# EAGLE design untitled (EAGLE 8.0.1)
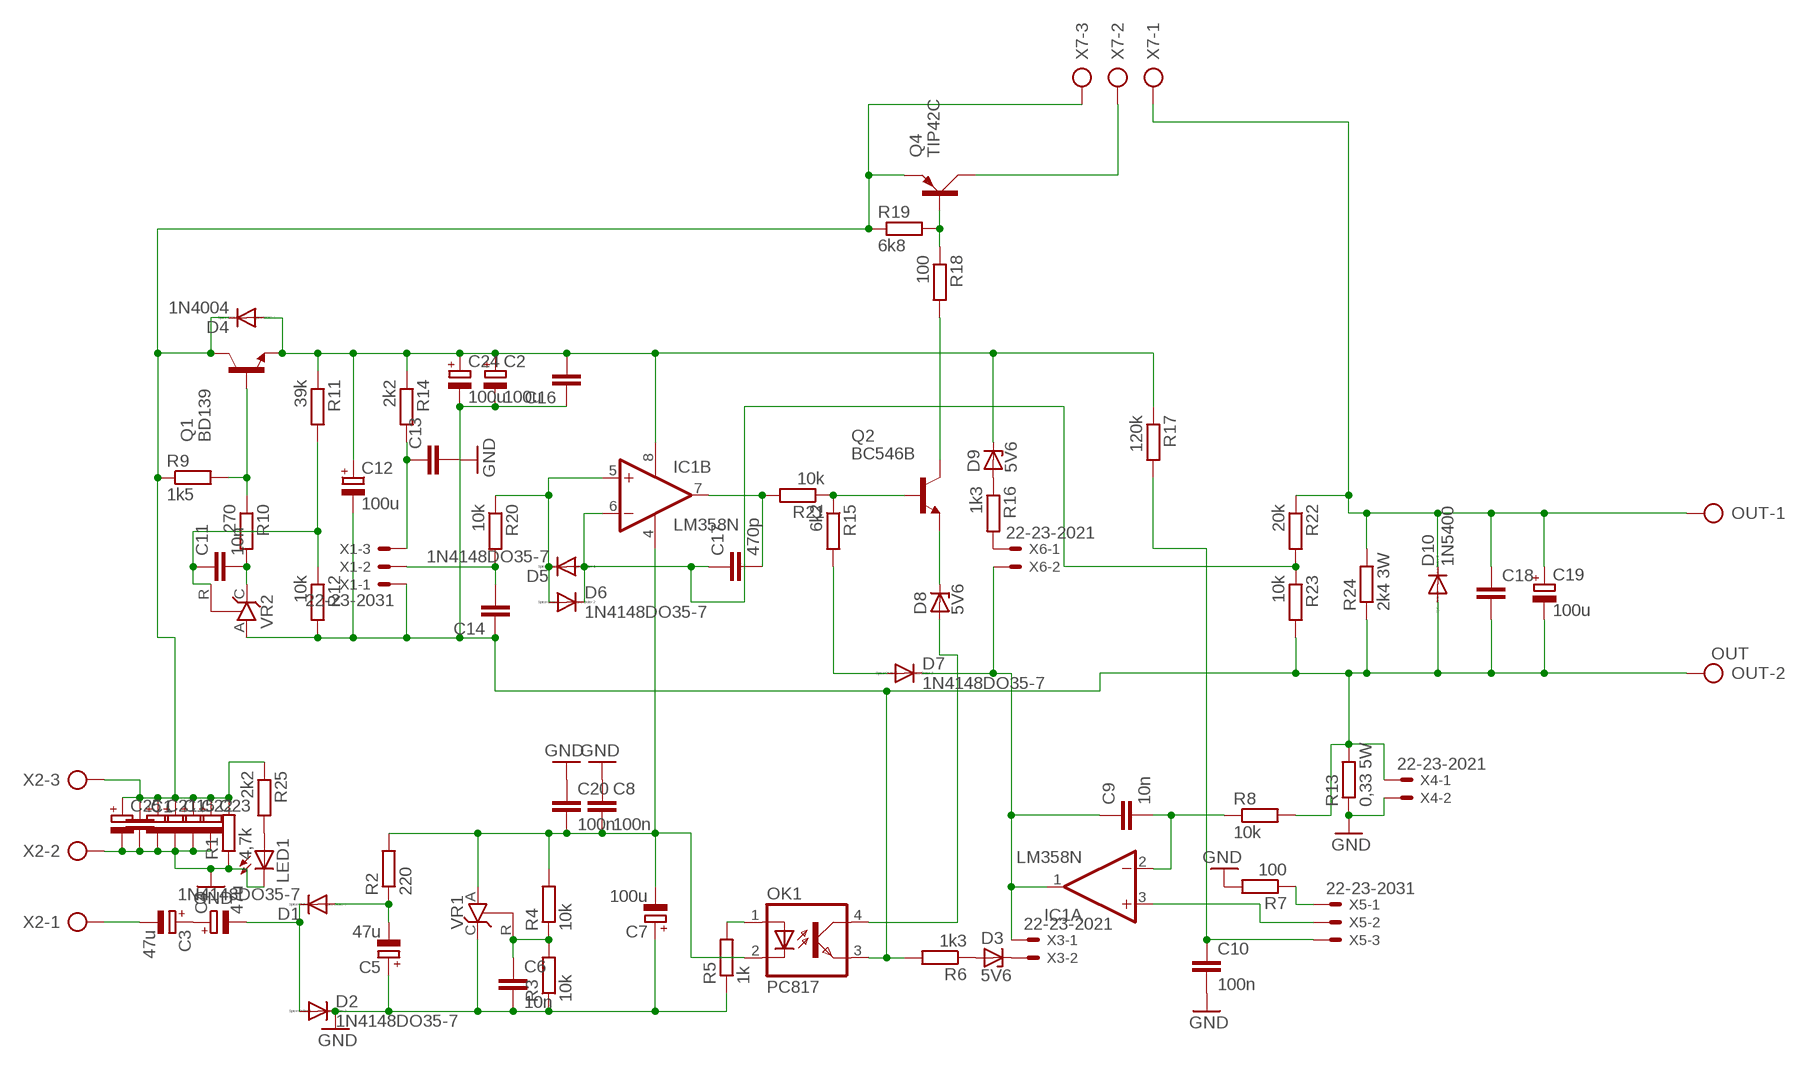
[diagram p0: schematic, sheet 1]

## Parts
C1  C-EU050-025X075  [C050-025X075]
C2  100u  CPOL-EUE2.5-7  [E2,5-7]
C3  47u  CPOL-EUE2.5-7  [E2,5-7]
C4  47u  CPOL-EUE2.5-7  [E2,5-7]
C5  47u  CPOL-EUE2.5-7  [E2,5-7]
C6  10n  C-EU050-025X075  [C050-025X075]
C7  100u  CPOL-EUE2.5-7  [E2,5-7]
C8  100n  C-EU050-025X075  [C050-025X075]
C9  10n  C-EU050-025X075  [C050-025X075]
C10  100n  C-EU050-025X075  [C050-025X075]
C11  10n  C-EU050-025X075  [C050-025X075]
C12  100u  CPOL-EUE2.5-7  [E2,5-7]
C13  C-EU050-025X075  [C050-025X075]
C14  C-EU050-025X075  [C050-025X075]
C15  CPOL-EUE5-10.5  [E5-10,5]
C16  C-EU050-025X075  [C050-025X075]
C17  470p  C-EU050-025X075  [C050-025X075]
C18  C-EU050-025X075  [C050-025X075]
C19  100u  CPOL-EUE2.5-7  [E2,5-7]
C20  100n  C-EU050-025X075  [C050-025X075]
C21  CPOL-EUE5-10.5  [E5-10,5]
C22  CPOL-EUE5-10.5  [E5-10,5]
C23  CPOL-EUE5-10.5  [E5-10,5]
C24  100u  CPOL-EUE2.5-7  [E2,5-7]
C25  CPOL-EUE5-10.5  [E5-10,5]
D1  1N4148DO35-7  [DO35-7]
D2  1N4148DO35-7  [DO35-7]
D3  5V6  BZD23  [SOD81]
D4  1N4004  [DO41-10]
D5  1N4148DO35-7  [DO35-7]
D6  1N4148DO35-7  [DO35-7]
D7  1N4148DO35-7  [DO35-7]
D8  5V6  BZD23  [SOD81]
D9  5V6  BZD23  [SOD81]
D10  1N5400  [DO201-15]
IC1  LM358N  [DIL08]
LED1  LED3MM  [LED3MM]
OK1  PC817  [DIL04]
OUT  OUT  AK300/2  [AK300/2]
Q1  BD139  [TO126]
Q2  BC546B  [TO92-EBC]
Q4  TIP42C  [TO220AV]
R1  4,7k  R-EU_0309/12  [0309/12]
R2  220  R-EU_0207/2V  [0207/2V]
R3  10k  R-EU_0207/7  [0207/7]
R4  10k  R-EU_0207/2V  [0207/2V]
R5  1k  R-EU_0207/7  [0207/7]
R6  1k3  R-EU_0207/7  [0207/7]
R7  100  R-EU_0207/7  [0207/7]
R8  10k  R-EU_0207/7  [0207/7]
R9  1k5  R-EU_0207/2V  [0207/2V]
R10  270  R-EU_0207/7  [0207/7]
R11  39k  R-EU_0207/7  [0207/7]
R12  10k  R-EU_0207/2V  [0207/2V]
R13  0,33 5W  R-EU_0922/22  [0922/22]
R14  2k2  R-EU_0207/2V  [0207/2V]
R15  6k2  R-EU_0207/2V  [0207/2V]
R16  1k3  R-EU_0207/2V  [0207/2V]
R17  120k  R-EU_0204/5  [0204/5]
R18  100  R-EU_0207/10  [0207/10]
R19  6k8  R-EU_0207/7  [0207/7]
R20  10k  R-EU_0207/2V  [0207/2V]
R21  10k  R-EU_0207/7  [0207/7]
R22  20k  R-EU_0207/10  [0207/10]
R23  10k  R-EU_0207/7  [0207/7]
R24  2k4 3W  R-EU_0309/12  [0309/12]
R25  2k2  R-EU_0207/2V  [0207/2V]
VR1  TL431CLP  [TO92-CLP]
VR2  TL431CLP  [TO92-CLP]
X1  22-23-2031  [22-23-2031]
X2  AK300/3  [AK300/3]
X3  22-23-2021  [22-23-2021]
X4  22-23-2021  [22-23-2021]
X5  22-23-2031  [22-23-2031]
X6  22-23-2021  [22-23-2021]
X7  AK300/3  [AK300/3]

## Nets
GND: C1.2 C5.+ C6.2 C7.+ C8.1 C10.2 C13.2 C15.- C20.1 C21.- C22.- C23.- C25.- D2.C LED1.K(C) R1.1 R3.1 R5.1 R7.2 R13.1 VR1.C X2.2 X4.2
N$1: C1.1 C15.+ C21.+ C22.+ C23.+ C25.+ D4.C Q1.2(C) Q4.E R1.2 R9.1 R19.1 R25.1 X2.3 X7.3
N$2: C7.- C8.2 C20.2 IC1.4(P:V-) OK1.2(C) R2.2 R4.2 VR1.A
N$3: C3.+ C4.+
N$4: C3.- X2.1
N$5: C4.- D1.C D2.A
N$6: C6.1 R3.2 R4.1 VR1.R
N$7: C5.- D1.A R2.1
N$8: C2.- C12.- C14.1 C16.1 C18.2 C19.- C24.- D10.A OK1.3(EMIT) OUT.2 R6.2 R8.2 R12.2 R13.2 R23.2 R24.1 VR2.A X1.1 X4.1
N$9: D3.A R6.1
N$10: OK1.1(A) R5.2
N$11: D3.C X3.2
N$12: C9.1 D7.C IC1.1(A:OUT) X3.1 X6.2
N$13: C9.2 IC1.2(A:-IN) R8.1
N$14: C10.1 R17.2 X5.3
N$15: IC1.3(A:+IN) X5.2
N$16: R7.1 X5.1
N$18: R16.2 X6.1
N$19: C2.+ C12.+ C16.2 C24.+ D4.A D9.C IC1.8(P:V+) Q1.1(E) R11.1 R14.1 R17.1
N$20: Q1.3(B) R9.2 R10.1
N$21: C11.2 R10.2 VR2.C
N$22: C11.1 R11.2 R12.1 VR2.R
N$24: C13.1 R14.2 X1.3
N$25: C14.2 R20.2 X1.2
N$26: D9.A R16.1
N$27: D5.C D6.A IC1.5(B:+IN) R20.1
N$29: C17.2 IC1.7(B:OUT) R21.2
N$30: Q2.B R15.1 R21.1
N$31: D7.A R15.2
N$32: D8.C Q2.E
N$33: D8.A OK1.4(COL)
N$37: Q4.B R18.1 R19.2
N$38: Q2.C R18.2
N$40: Q4.C X7.2
N$41: C18.1 C19.+ D10.C OUT.1 R22.1 R24.2 X7.1
N$42: C17.1 D5.A D6.C IC1.6(B:-IN) R22.2 R23.1
N$158: LED1.A R25.2

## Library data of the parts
C1 C6 C8-C11 C13 C14 C16-C18 C20 = resistor:C-EU: CAPACITOR, European symbol
C2-C5 C7 C12 C15 C19 C21-C25 = resistor:CPOL-EU: POLARIZED CAPACITOR, European symbol
D1 D2 D5-D7 = diode:1N4148: DIODE
D3 D8 D9 = diode:BZD23: Z DIODE
D4 = diode:1N4004: DIODE
D10 = diode:1N5400: DIODE
IC1 = linear:LM358: OP AMP also LM158; LM258; LM2904 Source: http://cache.national.com/ds/LM/LM158.pdf
LED1 = led:LED: LED
OK1 = optocoupler:PC817: SHARP OPTO COUPLER; MPN: PC817X4J000F; OC_FARNELL: 9707727; OC_NEWARK: 97K7059
OUT = con-ptr500:AK300/2: CONNECTOR; OC_FARNELL: unknown; OC_NEWARK: unknown
Q1 = transistor-npn:BD139*: NPN Transistor
Q2 = transistor-npn:BC546*: NPN Transistor
Q4 = transistor-power:TIP42C: PNP TRANSISTOR
R1-R25 = resistor:R-EU_: RESISTOR, European symbol
VR1 VR2 = v-reg:TL431CLP: VOLTAGE REGULATOR
X1 X5 = con-molex:22-23-2031: .100" (2.54mm) Center Header - 3 Pin; MF: MOLEX; MPN: 22-23-2031; OC_FARNELL: 1462950; OC_NEWARK: 30C0862
X2 X7 = con-ptr500:AK300/3: CONNECTOR; OC_FARNELL: unknown; OC_NEWARK: unknown
X3 X4 X6 = con-molex:22-23-2021: .100" (2.54mm) Center Header - 2 Pin; MF: MOLEX; MPN: 22-23-2021; OC_FARNELL: 1462926; OC_NEWARK: 25C3832

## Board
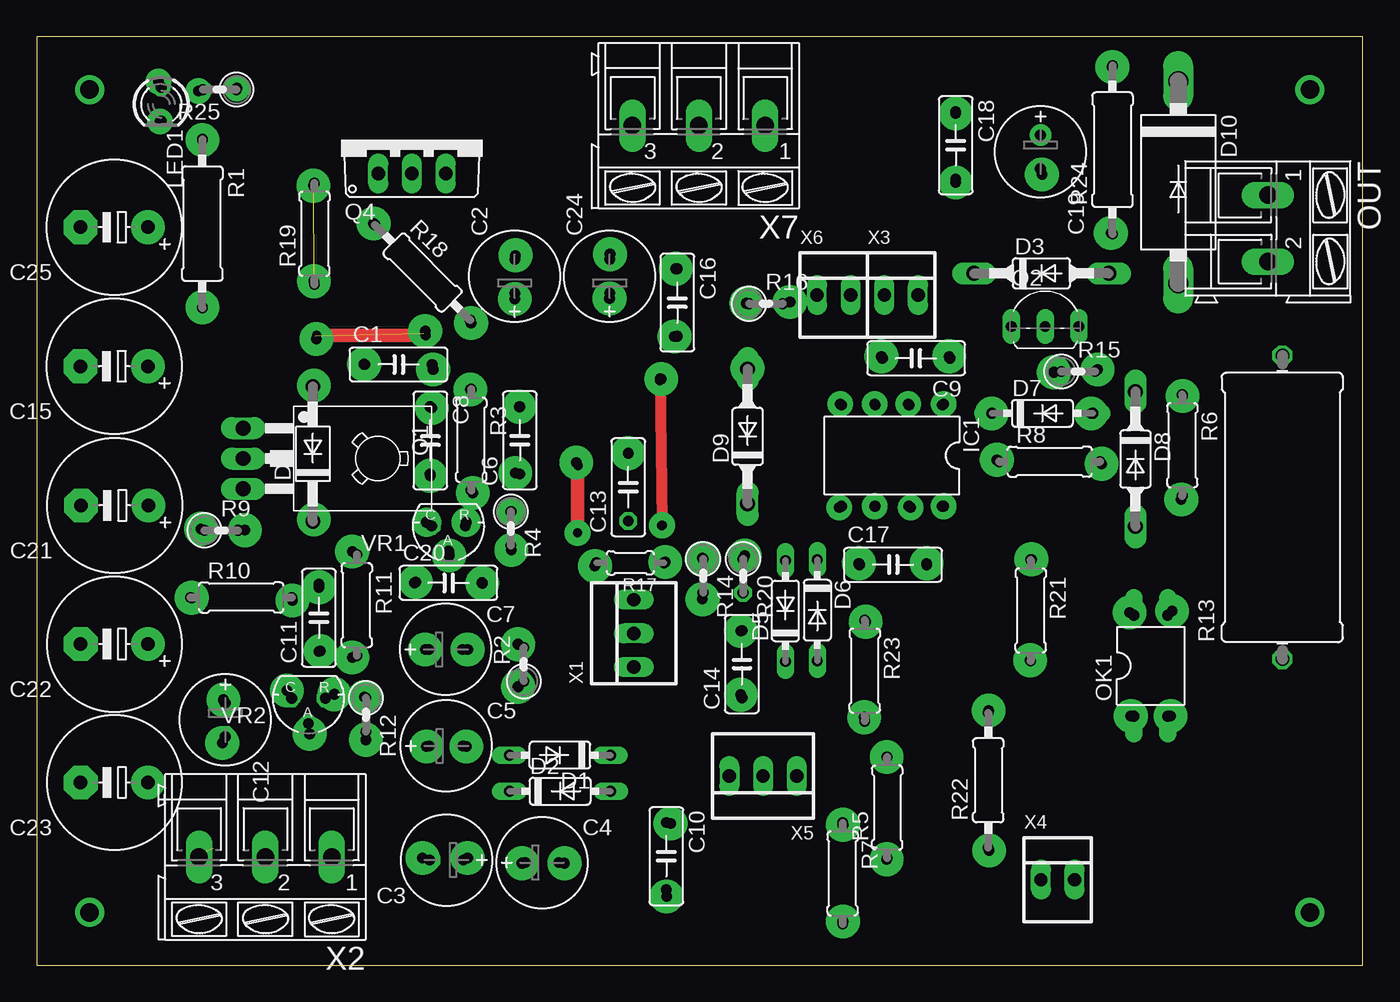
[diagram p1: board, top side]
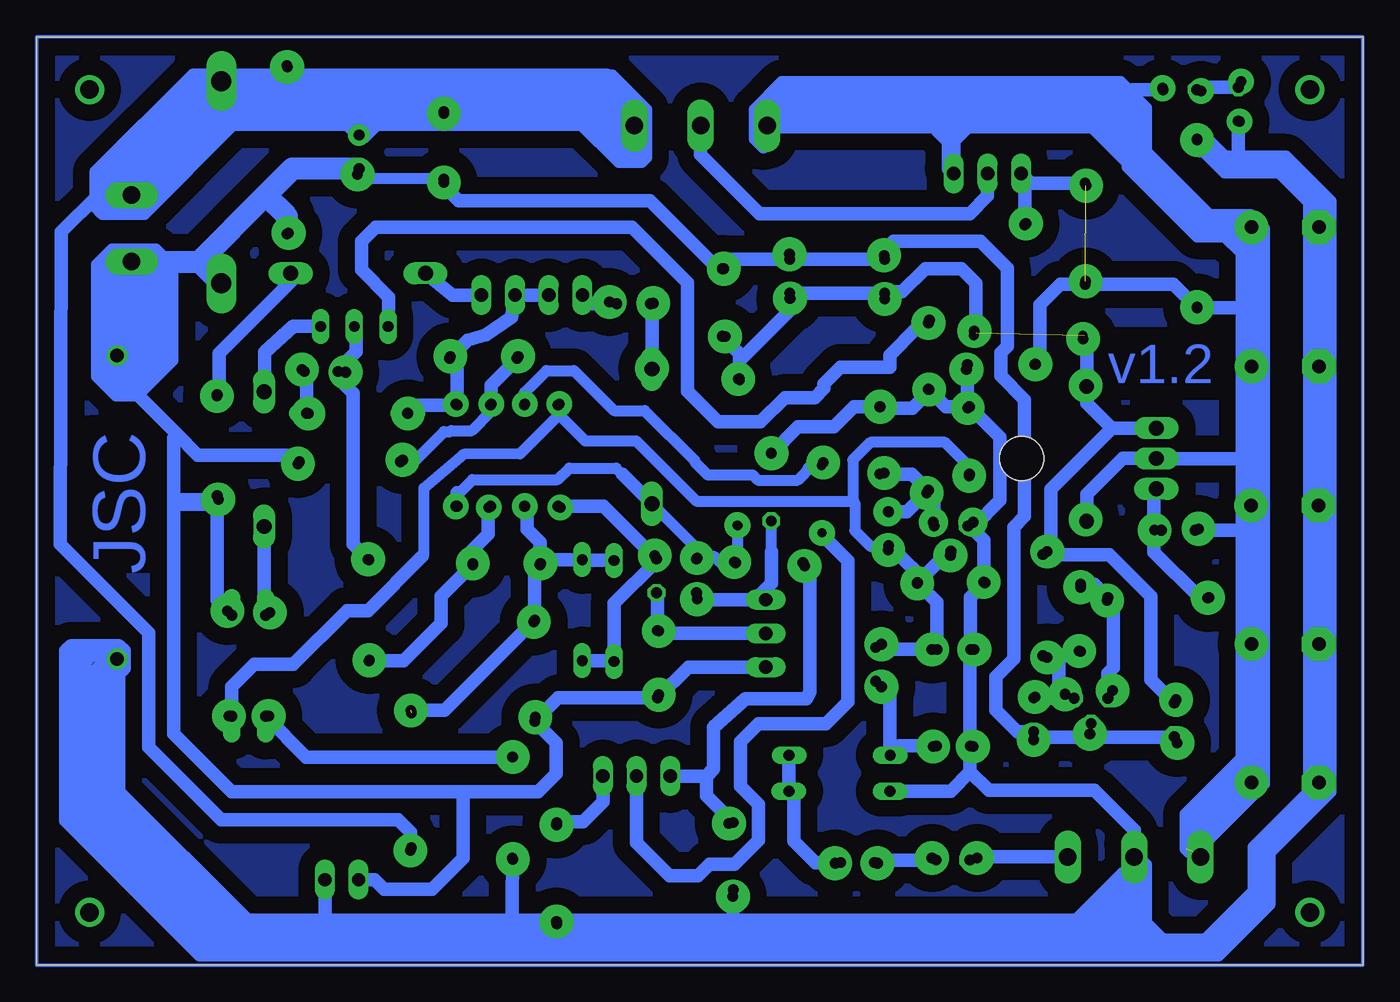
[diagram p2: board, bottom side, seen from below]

Size 100 x 70 mm. Coordinates in mm from the lower left corner, seen from the top.
Outline: 0,0 100,0 100,70 0,70 0,0
Copper layers (1*16): Top 0.035mm / dielectric 1.5mm / Bottom 0.035mm
Design rules "default": minimum track width 10mil, minimum drill 24mil, track to track 8mil, track to pad 8mil, pad to pad 8mil, via to via 8mil, smd to smd 8mil, copper to edge 40mil, drill to drill 8mil, minimum pad ring 10mil, minimum via ring 8mil, stop-mask expansion 4mil, vias tented up to drill 0mil, thermal gap 10mil

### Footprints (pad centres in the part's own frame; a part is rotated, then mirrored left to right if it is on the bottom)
C050-025X075 = drill 0.813 octagon: 1 -2.54,0; 2 2.54,0
E2,5-7 = drill 0.813 pad 1.6: + -1.27,0 | drill 0.813 pad 1.6 octagon: - 1.27,0
E5-10,5 = drill 1.016 pad 2.54: + -2.54,0 | drill 1.016 pad 2.54 octagon: - 2.54,0
DO35-7 = drill 0.813 long: A 3.81,0; C -3.81,0
SOD81 = drill 1.118 long: A 5.08,0; C -5.08,0
DO41-10 = drill 1.118: A 5.08,0; C -5.08,0
DO201-15 = drill 1.499 long: A 7.62,0; C -7.62,0
DIL08 = drill 0.813 pad 1.27: 1 -3.81,-3.81; 2 -1.27,-3.81; 3 1.27,-3.81; 4 3.81,-3.81; 5 3.81,3.81; 6 1.27,3.81; 7 -1.27,3.81; 8 -3.81,3.81
LED3MM = drill 0.813 octagon: A -1.27,0; K 1.27,0
DIL04 = drill 0.813 offset: 1 -1.27,-3.81; 2 1.27,-3.81; 3 1.27,3.81; 4 -1.27,3.81
AK300/2 = drill 1.321 long: 1 -2.515,0; 2 2.489,0
TO126 = drill 1.118 long: 1 -2.286,-5.08; 2 0,-5.08; 3 2.286,-5.08 | hole 3.302: 0,5.08
TO92-EBC = drill 0.813 long: B 0,-1.27; C -2.54,-1.27; E 2.54,-1.27
TO220AV = drill 1.016 long: B -2.54,-2.54; C 0,-2.54; E 2.54,-2.54
0309/12 = drill 0.813 octagon: 1 -6.35,0; 2 6.35,0
0207/2V = drill 0.813 octagon: 1 -1.27,0; 2 1.27,0
0207/7 = drill 0.813 octagon: 1 -3.81,0; 2 3.81,0
0922/22 = drill 1.016 octagon: 1 -11.43,0; 2 11.43,0
0204/5 = drill 0.813 octagon: 1 -2.54,0; 2 2.54,0
0207/10 = drill 0.813 octagon: 1 -5.08,0; 2 5.08,0
TO92-CLP = drill 0.813 octagon: A 0,1.905; C 1.27,0; R -1.27,0
22-23-2031 = drill 1 long: 1 -2.54,0; 2 0,0; 3 2.54,0
AK300/3 = drill 1.321 long: 1 -5.004,0; 2 0,0; 3 5.004,0
22-23-2021 = drill 1 long: 1 -1.27,0; 2 1.27,0

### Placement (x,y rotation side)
C1  27.29,45.29 0 top
C2  36.05,51.93 90 top
C3  30.9,7.94 180 top
C4  38.11,7.75 0 top
C5  30.89,16.54 0 top
C6  36.44,39.57 90 top
C7  30.85,23.81 0 top
C8  29.68,39.56 270 top
C9  66.31,45.75 180 top
C10  47.48,8.23 270 top
C11  21.29,26.19 90 top
C12  14.23,18.5 270 top
C13  44.61,36.03 90 top
C14  53.18,22.7 90 top
C15  5.85,45.15 180 top
C16  48.31,49.95 270 top
C17  64.57,30.2 0 top
C18  69.3,61.81 270 top
C19  75.69,61.31 270 top
C20  31.05,28.83 0 top
C21  5.9,34.66 180 top
C22  5.87,24.21 180 top
C23  5.87,13.78 180 top
C24  43.21,51.94 90 top
C25  5.86,55.63 180 top
D1  39.46,15.84 180 top
D2  39.47,13.13 0 top
D3  75.76,52.16 0 top
D4  20.83,38.55 90 top
D5  56.46,26.71 90 top
D6  58.86,26.77 270 top
D7  75.83,41.61 0 top
D8  82.84,38.16 270 top
D9  53.61,39.87 90 top
D10  86.07,59.02 270 top
IC1  64.49,38.42 180 top
LED1  9.4,64.9 270 top
OK1  84,22.58 0 top
OUT  92.83,55.53 270 top
Q1  20.65,38.2 270 top
Q2  76.04,49.42 0 top
Q4  28.3,62.22 0 top
R1  12.5,55.9 270 top
R2  36.73,22.69 90 top
R3  32.77,39.61 270 top
R4  35.75,32.92 270 top
R5  64.13,11.89 90 top
R6  86.38,39.2 270 top
R7  60.77,6.93 270 top
R8  76.38,37.96 0 top
R9  13.93,32.79 0 top
R10  15.43,27.73 0 top
R11  24.14,27.15 270 top
R12  24.83,18.88 270 top
R13  93.92,34.52 90 top
R14  50.25,29.36 270 top
R15  78.53,44.76 0 top
R16  54.99,49.87 0 top
R17  44.76,30.34 180 top
R18  29.1,52.22 315 top
R19  20.95,55.14 90 top
R20  53.26,29.35 270 top
R21  74.95,26.75 270 top
R22  71.75,13.95 90 top
R23  62.44,22.21 270 top
R24  81.12,61.47 90 top
R25  13.8,66 180 top
VR1  31.06,33.11 180 top
VR2  20.5,20.13 180 top
X1  45.03,25.02 90 top
X2  17.25,8.17 180 top
X3  65.19,50.52 0 top
X4  76.99,6.46 0 top
X5  54.77,14.27 180 top
X6  60.11,50.52 0 top
X7  49.93,63.28 180 top

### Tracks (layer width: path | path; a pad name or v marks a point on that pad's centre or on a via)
GND
  Bottom 1.016: 29.62,14.59 28.22,13.19 20.26,13.19 17.25,10.18 X2.2 17.25,7.47 | C8.1 27.37,39.79 27.37,35.04 29.3,33.11 VR1.C 29.63,33.11 28.57,32.05 28.57,28.89 C20.1 29.58,27.76 C7.+ 29.62,23.77 C5.+ 29.62,14.59 | C8.1 31.45,42.1 R3.1 32.77,43.2 33.97,42 36.33,42 C6.2 | C6.2 36.44,42.09 | 17.25,7.47 17.25,5.27 21.23,1.29 47.42,1.29 | 61.02,1.29 47.42,1.29 | 64.49,1.29 61.02,1.29 | 78.49,1.29 64.49,1.29 | 78.49,1.29 84.59,1.29 95.11,12 95.17,21.84 R13.1 | C10.2 47.48,1.35 47.42,1.29 | R7.2 60.77,1.54 61.02,1.29 | R5.1 64.18,1.6 64.49,1.29 | 17.25,7.47 17.29,7.43 17.29,2.92 15.55,1.18 11.74,1.18 8.1,4.82 8.1,8.84 3.32,13.62 C23.- 3.32,27.29 C22.- 3.22,37.87 C21.- 3.17,47.99 | C1.2 29.83,42.25 C8.1 | D2.C 31.08,13.13 29.62,14.59 | C13.2 42.58,40.6 39.89,40.6 38.38,42.11 C6.2 | 3.17,47.99 3.17,48.58 C15.- | 3.17,47.99 3.06,48.1 C25.- 3.32,57.69 5.84,60.21 8.9,60.21 | 8.9,60.21 10.46,60.21 R1.1 | LED1.K 9.4,60.71 8.9,60.21 | X4.2 78.26,1.52 78.49,1.29
N$1
  Bottom 1.016: D4.C 20.83,35.49 18.09,38.23 15.6,38.23 Q1.2 8.49,38.2 8.25,38.44 | X2.3 11.98,8.44 11.98,10.25 8.4,13.83 C23.+ 8.4,27.29 C22.+ 8.3,32.62 | 18.79,64.58 24.62,64.58 | 24.79,64.41 24.62,64.58 | X7.3 43.63,64.58 31.01,64.58 | 31.01,64.58 24.62,64.58 | 8.25,38.44 C21.+ 8.3,37.87 8.3,32.62 | 8.25,38.44 8.25,48.58 C15.+ 8.26,49.6 | 8.26,49.6 8.21,51.15 8.21,55.44 C25.+ 8.55,55.48 12.21,55.48 16.84,60.11 16.84,61.32 18.79,63.27 18.79,64.58 | R9.1 8.47,32.79 8.3,32.62 | 8.26,49.6 8.31,49.55 R1.2 14.28,51.33 R19.1 22.82,51.33 24.35,49.8 24.35,45.69 C1.1 | R25.1 17.37,66 18.79,64.58 | 31.01,64.58 31.01,59.85 Q4.E 30.84,62.14 29.91,63.07 29.91,63.48 31.01,64.58
N$2
  Bottom 0.813: 70.94,30.82 70.81,30.95 70.81,35.96 67.82,38.52 63.55,38.54 60.18,41.91 IC1.4 60.68,41.56 58.64,39.52 54.8,39.52 50.26,34.98 38.43,34.98 | R4.2 35.83,31.57 37.12,31.57 38.31,32.76 38.31,34.86 38.43,34.98 | C8.2 29.68,37.59 31.51,39.42 37.14,39.42 38.46,38.1 38.46,35.01 38.43,34.98
  Bottom 1.016: R2.2 36.58,23.81 C7.- 32.12,27.36 C20.2 33.23,29.2 | VR1.A 31.21,31.2 33.23,29.2 | R4.2 34.98,30.95 33.23,29.2 | OK1.2 85.27,20.99 83.58,22.68 80.65,22.68 76.59,26.74 75.02,26.74 70.94,30.82
N$3
  Bottom 1.016: C3.+ 36.65,7.94 C4.+
N$4
  Bottom 1.016: X2.1 29.4,8.17 C3.-
N$5
  Bottom 1.016: C4.- 41.28,7.75 42.89,9.36 42.89,12.61 D2.A D1.C
N$6
  Bottom 1.016: VR1.R 32.33,35.36 R3.2 | R3.2 34,37.03 C6.1 36.18,36.77 | R4.1 34.38,34.19 R3.2
N$7
  Bottom 1.016: R2.1 35.65,20.34 D1.A 34.95,16.54 C5.-
N$8
  Bottom 0.406: R6.2 89.67,35.39 89.67,35.5
  Bottom 0.813: C18.2 74.92,59.27 C19.-
  Bottom 1.016: R6.2 86.38,27.5 OK1.3 | 20.68,17.19 VR2.A | X1.1 50.86,22.48 C14.1 60.68,20.16 R23.2 60.82,16.78 60.82,14.44 62.18,13.08 68.08,13.08 | C18.2 69.83,59.27 68.17,57.61 53.74,57.61 48.62,52.49 C16.1 47.59,53.21 C24.- C2.- 36.09,53.24 36.09,53.87 35.39,54.57 28.86,54.57 26.81,52.52 26.81,46.66 27.31,46.16 27.31,44.44 25.51,42.64 25.51,33.83 26.33,33.01 26.33,23.1 27.69,21.74 27.69,19.23 26.07,17.61 R12.2 24.41,17.19 20.68,17.19 | 89.39,40.01 87.84,38.46 80.69,38.46 R8.2 | 89.39,40.01 94.04,44.66 94.04,45.83 R13.2 | 89.39,40.01 89.67,39.73 89.67,35.5 89.67,17.47 85.28,13.08 68.08,13.08 | X4.1 74.53,6.46 73.8,5.73 70.18,5.73 67.83,8.08 67.83,12.83 68.08,13.08 | C12.- 14.27,17.19 20.68,17.19
  Bottom 1.676: C19.- 80.71,60.04 82.71,58.04 | 87.71,53.04 OUT.2 93.92,51.95 R13.2 | 87.71,53.04 D10.A | 87.71,53.04 82.71,58.04 | R24.1 81.12,56.45 82.71,58.04
N$9
  Bottom 1.016: D3.A 80.82,51.55 86.23,46.14 86.23,43.16 R6.1
N$10
  Bottom 1.016: R5.2 79.66,15.7 OK1.1
N$11
  Bottom 1.016: X3.2 68.65,50.52 D3.C
N$12
  Bottom 1.016: X6.2 63.81,50.52 64,49.86 64,50.23 X3.1 64.18,48.84 66.09,47.51 67.49,47.11 C9.1 68.3,45.2 IC1.1 71.4,42.23 D7.C
N$13
  Bottom 0.813: IC1.2 65.76,41.72 67.17,40.31 68.72,40.31 68.8,40.23 69.28,40.23 71.55,37.96 R8.1
  Bottom 1.016: C9.2 63.77,45.69 65.73,43.73 65.73,42.26 IC1.2
N$14
  Bottom 1.016: 47.71,11 C10.1 49.49,12.78 49.49,14.27 | R17.2 41.68,29.8 41.68,20.63 41.95,20.11 46.56,20.11 48.96,17.96 48.96,14.8 49.49,14.27 | 49.49,14.27 X5.3
N$15  (via drill 0.7 pad 1.93)
  Top 1.016: v40.79,32.6 40.79,37.72 | 40.79,37.83 40.79,37.72 | 40.79,37.72 v40.83,37.68
  Bottom 0.813: IC1.3 63.22,43.16 61.56,44.82 59.49,44.82 56.47,41.8 54.15,41.8 50.33,37.98 50.33,37.88 49.41,36.96 46.02,36.96 45.63,36.57 42.6,36.57 41.49,37.68
  Bottom 1.016: v40.79,32.6 40.77,32.58 40.77,32.45 38.83,30.51 38.83,19.86 40.47,18.22 45.59,18.22 46.94,16.87 46.94,13.5 45.59,12.15 45.59,9.44 47.39,7.64 49.28,7.64 50.15,6.77 52.28,6.77 54.77,9.26 X5.2 | v40.83,37.68 41.49,37.68 41.72,37.45
N$16
  Bottom 1.016: X5.1 57.31,12.32 58.79,10.84 60.67,10.84 R7.1
N$17  (via drill 0.7 pad 1.93, 0.8 pad 2.54)
  Top 1.016: v21.12,47.48 29.27,47.48 v29.3,47.51
  Bottom 1.016: 29.3,48.3 v29.3,47.8 | v29.3,47.8 v29.3,47.51 | v29.3,47.51 v29.3,47.8 | v29.3,47.8 29.3,48.3 | v29.3,47.51 v29.3,47.8 | v29.3,47.8 29.3,48.3
N$18
  Bottom 1.016: R16.2 58.19,49.87 X6.1
N$19  (via drill 0.7 pad 1.93)  (1 unrouted)
  Top 0.813: v47.01,44.26 47.14,33.41 v47.17,33.17
  Bottom 0.813: 68.3,35.62 68.12,35.62 67.14,36.6 60.71,36.6 59.83,37.48 56.3,37.48 55.83,37.01 | v46.99,44.08 46.88,44.16 v47.01,44.26 | v47.17,33.17 47.17,30.47 R17.1 48.42,30.34 48.91,30.83 50.05,30.83 R14.1 50.25,31.43 D9.C
  Bottom 1.016: 18.93,40.49 Q1.1 | 18.93,40.49 23.52,35.9 23.52,31.58 R11.1 19.13,30.96 15.99,27.82 15.99,21.53 C12.+ | D4.A 20.83,42.38 18.93,40.49 | IC1.8 68.3,35.62 | D9.C 55.83,37.01 | 20.83,44.55 D4.A | 29.42,47.38 29.17,47.63 29.17,51.39 30.29,52.51 32.99,52.51 34.75,50.75 35.96,50.75 C2.+ C24.+ 43.21,49.36 46.99,45.58 | D4.A 20.83,47.27 21.02,47.46 | 48.33,47.39 C16.2 46.99,46.09 46.99,45.58 | 46.99,45.58 v46.99,44.08
N$20
  Bottom 1.016: R10.1 12.35,27.73 15.75,31.13 15.75,32.79 | 15.75,32.79 15.75,35.73 Q1.3 | R9.2 15.75,32.79
N$21
  Bottom 1.016: C11.2 20.24,28.73 R10.2 18.83,27.32 18.83,22.43 19.23,22.03 VR2.C
N$22
  Bottom 1.016: R12.1 22.61,20.15 VR2.R 22.92,21.28 22.92,23.34 | C11.1 21.6,23.34 22.92,23.34 | 22.92,23.34 R11.2
N$23
  Bottom 1.27: 87.05,34.83 86.57,34.83 86.57,34.85 89.5,34.85 89.5,34.91
N$24
  Bottom 0.813: 44.58,31.18 44.58,33.46 C13.1
  Bottom 1.016: 45.82,27.56 X1.3 | 45.82,27.56 49.72,27.56 R14.2 | 44.58,31.18 44.58,28.8 45.82,27.56
N$25
  Bottom 1.016: X1.2 52.96,25.02 C14.2 53.18,28 R20.2
N$26
  Bottom 1.016: D9.A 53.61,49.76 R16.1
N$27
  Bottom 1.016: IC1.5 57.25,34.61 R20.1 53.26,30.47 56.45,27.28 D5.C 56.52,22.96 D6.A
N$28  (via drill 0.7 pad 1.68)
  other vias: 29.35,47.48
N$29
  Bottom 1.016: IC1.7 65.96,34.41 65.96,32.48 67.11,31.33 C17.2 69.5,27.81 69.5,25.77 72.33,22.94 R21.2
N$30
  Bottom 1.016: Q2.B 75.9,48.43 75.9,46.24 77.26,44.88 R15.1 77.26,44.25 76.12,43.11 76.12,31.73 R21.1
N$31
  Bottom 1.016: D7.A 79.64,44.6 R15.2
N$32
  Bottom 1.016: Q2.E 80.67,48.16 82.81,46.19 82.81,43.27 D8.C
N$33
  Bottom 1.016: D8.A 82.84,26.5 OK1.4
N$35  (via drill 0.7 pad 1.93)
  other vias: 47.14,33.14
N$36  (via drill 0.7 pad 1.93)
  other vias: 46.96,44.23
N$37
  Bottom 1.016: R19.2 25.03,58.95 Q4.B 25.5,59.42 R18.1
N$38
  Bottom 1.016: Q2.C 73.44,50.35 75.5,52.41 75.5,54.57 74.44,55.63 55.1,55.63 50.93,51.46 50.93,43.27 48.63,40.97 45.41,40.97 43.59,42.79 41.31,42.79 40.62,43.48 40.62,43.85 39.41,45.06 35.65,45.06 35.65,46 33.65,48 33.32,48 R18.2
N$39  (via drill 1.4 pad 2.18)
  other vias: 96,66
N$40
  Bottom 1.016: 50.05,63.16 X7.2 49.93,61.11 45.48,56.66 29.64,56.66 28.3,58 Q4.C
N$41
  Bottom 1.016: 69.18,64.23 C18.1 | OUT.1 95.36,58.05 98.14,55.27 98.21,31.73 91.56,25.08 91.56,16.45 86.08,10.97 72.73,10.97 71.78,10.02 71.78,8.9 R22.1
  Bottom 1.676: 81.65,64.58 86.3,64.58 | 81.65,64.58 77.31,64.58 75.69,62.96 C19.+ 73.92,64.35 C18.1 56,64.35 X7.1 | 86.3,64.58 OUT.1 | D10.C 86.07,64.81 86.3,64.58 | R24.2 81.12,65.11 81.65,64.58
N$42  (via drill 0.8 pad 2.54)  (1 unrouted)
  Bottom 1.016: C17.1 62.03,31.87 63.02,32.86 63.02,34.41 IC1.6 | D5.A 58.8,30.52 D6.C 61.65,30.58 C17.1 | 62.5,25.96 R23.1 | R23.1 62.44,29.79 C17.1 | v71.78,19.21 69.25,19.21 R23.1
N$43  (via drill 1.4 pad 2.18)
  other vias: 4,66
N$44  (via drill 1.4 pad 2.18)
  other vias: 4,4
N$45  (via drill 1.4 pad 2.18)
  other vias: 96,4
N$46  (via drill 0.8 pad 2.54)  (1 unrouted)
  other vias: 20.92,51.56 20.88,58.76
N$47  (via drill 0.8 pad 2.54)
  other vias: 12.5,49.6
N$48  (via drill 0.8 pad 2.54)
  other vias: 12.5,62.2
N$49  (via drill 0.8 pad 2.54)
  other vias: 25.41,55.92
N$50  (via drill 0.8 pad 2.54)
  other vias: 21.1,47.2
N$51  (via drill 0.8 pad 2.54)
  other vias: 20.9,43.7
N$52  (via drill 0.8 pad 2.54)
  other vias: 24.7,45.3
N$53  (via drill 0.8 pad 2.54)
  other vias: 29.9,44.9
N$54  (via drill 0.8 pad 2.54)
  other vias: 29.8,42
N$55  (via drill 0.8 pad 2.54)
  other vias: 32.7,43.4
N$56  (via drill 0.8 pad 2.54)
  other vias: 36.4,42.1
N$57  (via drill 0.8 pad 2.54)
  other vias: 29.7,36.9
N$58  (via drill 0.8 pad 2.54)
  other vias: 20.9,33.6
N$59  (via drill 0.8 pad 2.54)
  other vias: 12.4,32.9
N$60  (via drill 0.8 pad 2.54)
  other vias: 15.7,32.8
N$61  (via drill 0.8 pad 2.54)
  other vias: 11.7,27.7
N$62  (via drill 0.8 pad 2.54)
  other vias: 19.3,27.5
N$63  (via drill 0.8 pad 2.54)
  other vias: 21.3,28.5
N$64  (via drill 0.8 pad 2.54)
  other vias: 21.4,23.7
N$65  (via drill 0.8 pad 2.54)
  other vias: 23.8,23.2
N$66  (via drill 0.8 pad 2.54)
  other vias: 23.8,31.2
N$67  (via drill 0.8 pad 2.54)
  other vias: 14,16.76
N$68  (via drill 0.8 pad 2.54)
  other vias: 14.09,20.02
N$69  (via drill 0.8 pad 2.54)
  other vias: 20.59,17.45
N$70  (via drill 0.8 pad 2.54)
  other vias: 18.87,20.71
N$71  (via drill 0.8 pad 2.54)
  other vias: 22.45,20.43
N$72  (via drill 0.8 pad 2.54)
  other vias: 24.73,20.22
N$73  (via drill 0.8 pad 2.54)
  other vias: 24.82,17
N$74  (via drill 0.8 pad 2.54)
  other vias: 29.1,8.1
N$75  (via drill 0.8 pad 2.54)
  other vias: 32.5,8.1
N$76  (via drill 0.8 pad 2.54)
  other vias: 36.6,7.7
N$77  (via drill 0.8 pad 2.54)
  other vias: 39.8,7.7
N$78  (via drill 0.8 pad 2.54)
  other vias: 47.5,5.2
N$79  (via drill 0.8 pad 2.54)
  other vias: 47.8,10.7
N$80  (via drill 0.8 pad 2.54)
  other vias: 60.8,3.3
N$81  (via drill 0.8 pad 2.54)
  other vias: 60.8,10.6
N$82  (via drill 0.8 pad 2.54)
  other vias: 64.1,8
N$83  (via drill 0.8 pad 2.54)
  other vias: 64.1,15.7
N$84  (via drill 0.8 pad 2.54)
  other vias: 62.4,18.7
N$85  (via drill 0.8 pad 2.54)
  other vias: 71.82,8.65
N$86  (via drill 0.8 pad 2.54)
  other vias: 32.4,16.5
N$87  (via drill 0.8 pad 2.54)
  other vias: 29.4,16.5
N$88  (via drill 0.8 pad 2.54)
  other vias: 32.5,23.8
N$89  (via drill 0.8 pad 2.54)
  other vias: 36.3,24.2
N$90  (via drill 0.8 pad 2.54)
  other vias: 36.3,21
N$91  (via drill 0.8 pad 2.54)
  other vias: 29.3,23.8
N$92  (via drill 0.8 pad 2.54)
  other vias: 28.6,28.9
N$93  (via drill 0.8 pad 2.54)
  other vias: 33.6,28.8
N$94  (via drill 0.8 pad 2.54)
  other vias: 31.1,30.9
N$95  (via drill 0.8 pad 2.54)
  other vias: 35.8,31.3
N$96  (via drill 0.8 pad 2.54)
  other vias: 32.9,35.6
N$97  (via drill 0.8 pad 2.54)
  other vias: 36.1,37.1
N$98  (via drill 0.8 pad 2.18)
  other vias: 35.8,34.2
N$99  (via drill 0.8 pad 2.18)
  other vias: 32.4,33.4
N$100  (via drill 0.8 pad 2.18)
  other vias: 29.4,33.4
N$101  (via drill 0.8 pad 2.54)
  other vias: 32.76,48.42
N$102  (via drill 0.8 pad 2.54)
  other vias: 36.06,50.23
N$103  (via drill 0.8 pad 2.54)
  other vias: 36.11,53.51
N$104  (via drill 0.8 pad 2.54)
  other vias: 43.24,53.6
N$105  (via drill 0.8 pad 2.54)
  other vias: 43.2,50.25
N$106  (via drill 0.8 pad 2.54)
  other vias: 56.8,50
N$107  (via drill 0.8 pad 2.54)
  other vias: 53.5,49.9
N$108  (via drill 0.8 pad 2.54)
  other vias: 53.6,45
N$109  (via drill 0.8 pad 2.54)
  other vias: 47.1,44.2
N$110  (via drill 0.8 pad 2.54)
  other vias: 48.1,47.4
N$111  (via drill 0.8 pad 2.54)
  other vias: 48.2,52.5
N$112  (via drill 0.8 pad 2.54)
  other vias: 40.7,37.9
N$113  (via drill 0.8 pad 2.54)
  other vias: 44.6,38.6
N$114  (via drill 0.8 pad 2.54)
  other vias: 42.1,30.1
N$115  (via drill 0.8 pad 2.54)
  other vias: 47.4,30.4
N$116  (via drill 0.8 pad 2.54)
  other vias: 50.2,30.7
N$117  (via drill 0.8 pad 2.54)
  other vias: 50.2,27.6
N$118  (via drill 0.8 pad 2.54)
  other vias: 53.4,30.9
N$119  (via drill 0.8 pad 2.54)
  other vias: 53.1,25.2
N$120  (via drill 0.8 pad 2.54)
  other vias: 53.1,20.4
N$121  (via drill 0.8 pad 2.54)
  other vias: 85.5,18.8
N$122  (via drill 0.8 pad 2.54)
  other vias: 82.5,18.8
N$123  (via drill 0.8 pad 2.54)
  other vias: 85.6,26.7
N$124  (via drill 0.8 pad 2.54)
  other vias: 82.4,26.6
N$125  (via drill 0.8 pad 2.54)
  other vias: 74.9,23
N$126  (via drill 0.8 pad 2.54)
  other vias: 75,30.6
N$127  (via drill 0.8 pad 2.54)
  other vias: 67.1,30.3
N$128  (via drill 0.8 pad 2.54)
  other vias: 62,30.3
N$129  (via drill 0.8 pad 2.54)
  other vias: 62.5,25.9
N$130  (via drill 0.8 pad 2.54)
  other vias: 63.7,45.9
N$131  (via drill 0.8 pad 2.54)
  other vias: 68.8,45.9
N$132  (via drill 0.8 pad 2.54)
  other vias: 72,41.6
N$133  (via drill 0.8 pad 2.54)
  other vias: 79.5,41.6
N$134  (via drill 0.8 pad 2.54)
  other vias: 80,44.9
N$135  (via drill 0.8 pad 2.54)
  other vias: 76.7,44.7
N$136  (via drill 0.8 pad 2.54)
  other vias: 86.4,42.9
N$137  (via drill 0.8 pad 2.54)
  other vias: 86.3,35.1
N$138  (via drill 0.8 pad 2.54)
  other vias: 80.3,37.8
N$139  (via drill 0.8 pad 2.54)
  other vias: 72.4,38.1
N$140  (via drill 0.8 pad 2.54)
  other vias: 81,55.2
N$141  (via drill 0.8 pad 2.54)
  other vias: 81.1,67.7
N$142  (via drill 0.8 pad 2.54)
  other vias: 69.3,59
N$143  (via drill 0.8 pad 2.54)
  other vias: 69.3,64.2
N$144  (via drill 0.8 pad 2.54)
  other vias: 75.8,59.6
N$145  (via drill 0.8 pad 1.93)
  other vias: 60.6,42.3
N$146  (via drill 0.8 pad 1.93)
  other vias: 63.2,42.3
N$147  (via drill 0.8 pad 1.93)
  other vias: 65.7,42.3
N$148  (via drill 0.8 pad 1.93)
  other vias: 68.4,42.3
N$149  (via drill 0.8 pad 1.93)
  other vias: 60.5,34.5
N$150  (via drill 0.8 pad 1.93)
  other vias: 63.2,34.6
N$151  (via drill 0.8 pad 1.93)
  other vias: 65.9,34.5
N$152  (via drill 0.8 pad 1.93)
  other vias: 68.4,34.6
N$153
  Bottom 1.016: 18.1,6.9 21.6,3.4 84.1,3.4 93.8,13.1 93.8,22 93.4,22.4 93.4,23.7 93.8,24.1 97.4,24.1 97.8,23.7 97.8,10.9 87.7,0.8 10.9,0.8 7.1,4.6 7.1,8.5 2.5,13.1 2.5,57.6 5.8,60.9 10.4,60.9 11.5,62 11.7,62 12.3,61.4 12,61.4 10.4,59.8 6.3,59.8 4,57.5 4,13.1 8.2,8.9 8.2,5.6 11.9,1.9 15.1,1.9 16.4,3.2 16.4,7.6 17.2,8.4 17.2,7.6 19,5.8 18.4,5.8 17.9,6.3 17.9,2.9 16.5,1.5 20.3,1.5 20.4,1.4 20.1,1.4 18.2,3.3 18.2,2.7 17.8,2.3 18.7,2.3 19.1,1.9 18.2,1.9 17.7,2.4 17.7,4.6 18.2,5.1 18.3,5.1 | 18.3,5.1 18.7,5.1 21.9,1.9 87.6,1.9 97.2,11.5 97.2,11.3 87.4,1.5 85.5,1.5 85,1 85.6,1 86.9,2.3 87.4,2.3 97.2,12.1 97.2,23.1 96.9,23.4 95.8,23.4 | 94.1,23.4 95.8,23.4 | 95.8,23.4 96.6,22.6 96.6,12.1 96.5,12 96.5,21.3 94.9,22.9 94.9,22.3 95.9,21.3 95.9,11.9 86.6,2.6 86.6,3.9 95.5,12.8 95.5,20.6 94.3,21.8 94.3,12.6 84.6,2.9 84.6,2.6 84.8,2.4 85.1,2.4 86.4,3.7 | 84.3,2.7 20.7,2.7 18.3,5.1
N$154  (1 unrouted)
  Bottom 1.016: 12.8,8.6 12.2,8.6 11.8,8.2 11.8,9.4 7.5,13.7 7.5,55.5 8.5,56.5 11.6,56.5 16.4,61.3 16.4,64.6 18.3,66.5 43.8,66.5 45.8,64.5 45.8,62.3 45.2,61.7 | 23.9,64.1 24.3,63.7 | 23.9,64.1 24,64.1 | 25.3,63.7 25.2,63.8 26.7,63.8 | 44.8,62.4 45.2,62.8 44.7,62.8 43.6,63.9 30.7,63.9 | 30.7,63.9 30.4,64.2 30.4,64.1 31.3,63.2 | 31.3,63.2 32.02,63.2 | 32.02,63.2 44.1,63.2 44.6,62.7 44.6,63.1 45.2,63.7 45.2,64.1 43.6,65.7 18.5,65.7 17,64.2 17,62.4 17.2,62.2 17.2,63.6 17.8,64.2 17.8,63.2 18.1,62.9 18.1,64.6 18.5,65 43.2,65 43.4,65.2 | 26.7,63.8 26.7,63.7 | 31.3,63.2 20.4,63.2 17.7,60.5 17.7,60.2 12.5,55 10.4,55 9.1,53.7 9.1,15.6 13.3,11.4 13.3,8.8 12.6,8.1 12.6,11 8.8,14.8 8.8,13.7 12.8,9.7 12.8,10.4 8.4,14.8 8.4,54 9.4,55 10.8,55 14.8,59 15.1,59 19.7,63.6 19.7,63.9 23.7,63.9 23.9,64.1 | 30.7,63.9 30.6,63.8 26.7,63.8 | 32.05,62.88 32.05,63.9 | 32.05,62.88 31.26,62.09 31.26,60.04 31.02,59.8 | 32.02,63.2 32.02,62.91 32.05,62.88
N$156
  Bottom 1.016: 54.8,65 54.9,65 57,67.1 88.2,67.1 95.5,59.8 95.5,57.2 95,56.7 91.9,56.7 85.2,63.4 58.9,63.4 56.1,60.6 54.4,60.6 54.1,60.9 54.1,64.5 56.6,67 56.6,64.3 54.5,62.2 54.5,61.6 54.8,61.3 56.4,61.3 58.3,63.2 56.1,63.2 54.9,62 56.1,62 57.5,63.4 57.5,62.8 56.3,61.6 56.3,65.1 55.8,65.6 56.4,65.6 57.1,66.3 88.1,66.3 94.9,59.5 94.9,57.4 92.5,57.4 85.9,64 58.3,64 57.1,65.2 88.1,65.2 94.2,59.1 94.2,58.7 94,58.5 93.8,58.5 87.3,65 87.3,65.2 87.9,65.8 56.8,65.8 56.7,65.7 73.9,65.7 75.4,64.2 75.4,64.8 75.6,64.8 75.9,64.5
N$157
  Bottom 1.016: 92.9,43 94,43 95.4,44.4 95.4,52.8 94.3,53.9 91,53.9 89.8,52.7 89.8,45.6 92.4,43 93.1,43 94.6,44.5 94.6,52.4 93.8,53.2 91.4,53.2 90.3,52.1 90.3,46.3 92.4,44.2 92.6,44.2 93.3,44.9 93.3,51.1 92.4,52 91.4,52 91.2,51.8 91.2,46.7 92.8,45.1 92.8,50.7 92,51.5 92,46.8 92.4,46.4
N$158
  Bottom 1.016: LED1.A 12.36,66.17 R25.2
N$159  (via drill 0.8 pad 1.93)
  other vias: 9.3,63.6
N$160  (via drill 0.8 pad 1.93)
  other vias: 9.2,66.6
N$161  (via drill 0.8 pad 1.93)
  other vias: 12.2,65.9
N$162  (via drill 0.8 pad 1.93)
  other vias: 15.1,66.1
N$163
  pour Bottom (isolate 1.27): 0.5,69.5 99.5,69.5 99.5,0.5 0.5,0.5
N$164
  Bottom 0.254: 0,0 100,0 100,70 0,70 0,0

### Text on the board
Bottom: v1.2 | JSC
